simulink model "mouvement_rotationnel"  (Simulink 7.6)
settings: Solver=ode15s  StartTime=0.0  StopTime=1.5  RelTol=1e-3
StopFcn:
  | close all
  | load vitesse_position.mat
  | plot(x(1,:),x(2,:),x(1,:),x(3,:))
  | axis([0 1.5 0 125])
  | grid
  | title('Position et vitesse angulaires')
  | delete *.mat
undefined symbols (not defined in the file or in its folder): sigbuilder_block
libraries: fl_lib x8, nesl_utility x5, elec_lib x1

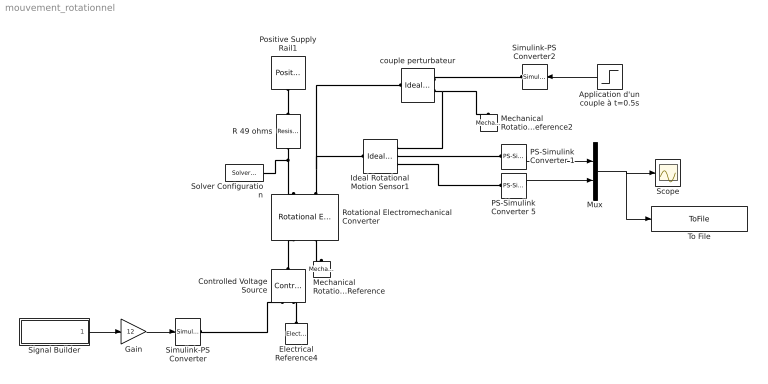
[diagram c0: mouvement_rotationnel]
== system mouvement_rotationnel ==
  Application d'un couple à t=0.5s : Step  Time=0.5  After=-15e-3  SampleTime=0
  Controlled Voltage Source : fl_lib/Electrical/Electrical Sources/Controlled Voltage Source  DialogController=NetworkEngine.DynNeDlgSource  SystemSampleTime=-1  i_Log=off  v_Log=off  LocalVarNames=|i|v  LocalVarDescs=|i|v  LocalVarLogging=[0 0]
  Electrical Reference4 : fl_lib/Electrical/Electrical Elements/Electrical Reference  DialogController=NetworkEngine.DynNeDlgSource  SystemSampleTime=-1  i_Log=off  LocalVarNames=|i  LocalVarDescs=|i  LocalVarLogging=[]
  Gain : Gain  Gain=12
  Ideal Rotational Motion Sensor1 : fl_lib/Mechanical/Mechanical Sensors/Ideal Rotational Motion Sensor  DialogController=NetworkEngine.DynNeDlgSource  SystemSampleTime=-1  offset=0 rad  w_Log=off  t_Log=off  phi_Log=off  LocalVarNames=|w|t|phi  LocalVarDescs=|w|t|phi  LocalVarLogging=[0 0 0]
  Mechanical Rotational Reference : fl_lib/Mechanical/Rotational Elements/Mechanical Rotational Reference  DialogController=NetworkEngine.DynNeDlgSource  SystemSampleTime=-1  t_Log=off  LocalVarNames=|t  LocalVarDescs=|t  LocalVarLogging=[]
  Mechanical Rotational Reference2 : fl_lib/Mechanical/Rotational Elements/Mechanical Rotational Reference  DialogController=NetworkEngine.DynNeDlgSource  SystemSampleTime=-1  t_Log=off  LocalVarNames=|t  LocalVarDescs=|t  LocalVarLogging=[]
  Mux : Mux  Inputs=2
  PS-Simulink Converter 1 : nesl_utility/PS-Simulink Converter  DialogController=NetworkEngine.DynNeUtilDlgSource  SystemSampleTime=-1  PhysicalDomain=network_engine_domain  LeftPortType=input  RightPortType=output  SubClassName=ps_output  Unit=rad/s  AffineConversion=off
  PS-Simulink Converter 5 : nesl_utility/PS-Simulink Converter  DialogController=NetworkEngine.DynNeUtilDlgSource  SystemSampleTime=-1  PhysicalDomain=network_engine_domain  LeftPortType=input  RightPortType=output  SubClassName=ps_output  Unit=rad  AffineConversion=off
  Positive Supply Rail1 : elec_lib/Sources/Positive Supply Rail  DialogController=NetworkEngine.DynNeDlgSource  SystemSampleTime=-1  v0=12 V  current_Log=off  voltage_Log=off  power_Log=off  LocalVarNames=|current|voltage|power  LocalVarDescs=|Current (A)|Voltage (V)|Power (W)  LocalVarLogging=[0 0 0]
  R 49 ohms : fl_lib/Electrical/Electrical Elements/Resistor  DialogController=NetworkEngine.DynNeDlgSource  SystemSampleTime=-1  R=49 Ohm  i_Log=off  v_Log=off  LocalVarNames=|i|v  LocalVarDescs=|i|v  LocalVarLogging=[0 0]
  Rotational Electromechanical Converter : fl_lib/Electrical/Electrical Elements/Rotational Electromechanical Converter  DialogController=NetworkEngine.DynNeDlgSource  SystemSampleTime=-1  K=0.1 V/(rad/s)  i_Log=off  v_Log=off  t_Log=off  w_Log=off  LocalVarNames=|i|v|t|w  LocalVarDescs=|i|v|t|w  LocalVarLogging=[0 0 0 0]
  Scope : Scope
  Signal Builder : Subsystem  Tag=STV Subsys  LoadFcn=sigbuilder_block('load');  StartFcn=sigbuilder_block('start');  StopFcn=sigbuilder_block('stop');  ClipboardFcn=sigbuilder_block('clipboard');
  Simulink-PS Converter : nesl_utility/Simulink-PS Converter  DialogController=NetworkEngine.DynNeUtilDlgSource  SystemSampleTime=-1  PhysicalDomain=network_engine_domain  LeftPortType=input  RightPortType=output  SubClassName=ps_input  Unit=1  AffineConversion=off  InputFilterTimeConstant=.001  UdotUserProvided=0
  Simulink-PS Converter2 : nesl_utility/Simulink-PS Converter  DialogController=NetworkEngine.DynNeUtilDlgSource  SystemSampleTime=-1  PhysicalDomain=network_engine_domain  LeftPortType=input  RightPortType=output  SubClassName=ps_input  Unit=1  AffineConversion=off  InputFilterTimeConstant=.001  UdotUserProvided=0
  Solver Configuration : nesl_utility/Solver Configuration  DialogController=NetworkEngine.DynNeUtilDlgSource  SystemSampleTime=-1  PhysicalDomain=network_engine_domain  LeftPortType=input  RightPortType=generic  SubClassName=solver  Accelerate=off  Profile=off  ResidualTolerance=1e-9  MaxNonlinIter=12  MaxModeIter=2  DoFixedCost=off  UseLocalSampling=off  DoDC=off  LinearAlgebra=Sparse  LocalSolverSampleTime=.001  LocalSolverChoice=NE_BACKWARD_EULER_ADVANCER  UseLocalSolver=off
  To File : ToFile  Filename=vitesse_position  MatrixName=x
  couple perturbateur : fl_lib/Mechanical/Mechanical Sources/Ideal Torque Source  DialogController=NetworkEngine.DynNeDlgSource  SystemSampleTime=-1  w_Log=off  t_Log=off  LocalVarNames=|torque|rel_velocity|power  LocalVarDescs=|Torque (N*m)|Relative velocity (rad/s)|Power generated by the source (W)  LocalVarLogging=[0 0 0]
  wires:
  PS-Simulink Converter 5/1 -> Mux/2
  Mux/1 -> Scope/1, To File/1
  PS-Simulink Converter 1/1 -> Mux/1
  Application d'un couple à t=0.5s/1 -> Simulink-PS Converter2/1
  Gain/1 -> Simulink-PS Converter/1
  Signal Builder/1(Signal 2) -> Gain/1
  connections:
  Ideal Rotational Motion Sensor1/RConn3 -- PS-Simulink Converter 5/LConn1
  Rotational Electromechanical Converter/RConn2 -- Mechanical Rotational Reference/LConn1
  Rotational Electromechanical Converter/LConn2 -- Ideal Rotational Motion Sensor1/LConn1 -- couple perturbateur/LConn1
  Ideal Rotational Motion Sensor1/RConn2 -- PS-Simulink Converter 1/LConn1
  couple perturbateur/RConn2 -- Mechanical Rotational Reference2/LConn1 -- Ideal Rotational Motion Sensor1/RConn1
  couple perturbateur/RConn1 -- Simulink-PS Converter2/RConn1
  R 49 ohms/RConn1 -- Rotational Electromechanical Converter/LConn1 -- Solver Configuration/RConn1
  Simulink-PS Converter/RConn1 -- Controlled Voltage Source/RConn1
  Electrical Reference4/LConn1 -- Controlled Voltage Source/RConn2
  Controlled Voltage Source/LConn1 -- Rotational Electromechanical Converter/RConn1
  Positive Supply Rail1/RConn1 -- R 49 ohms/LConn1

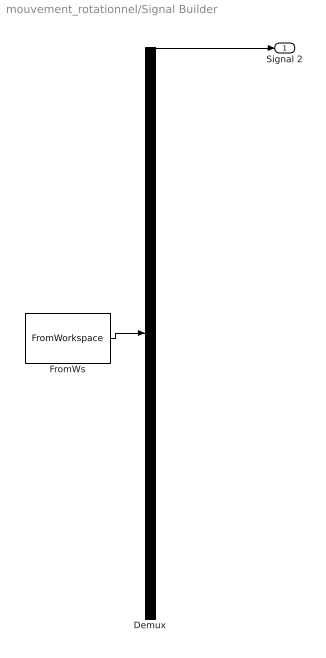
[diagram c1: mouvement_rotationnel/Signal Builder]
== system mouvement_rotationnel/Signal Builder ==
  Demux : Demux  Tag=STV Demux  Outputs=1
  FromWs : FromWorkspace  Tag=STV FromWs  VariableName=tuvar  SampleTime=0  SigBuilderData=DataTag0  VnvData=DataTag1
  Signal 2 : Outport  Tag=STV Outport
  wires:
  FromWs/1 -> Demux/1
  Demux/1 -> Signal 2/1
